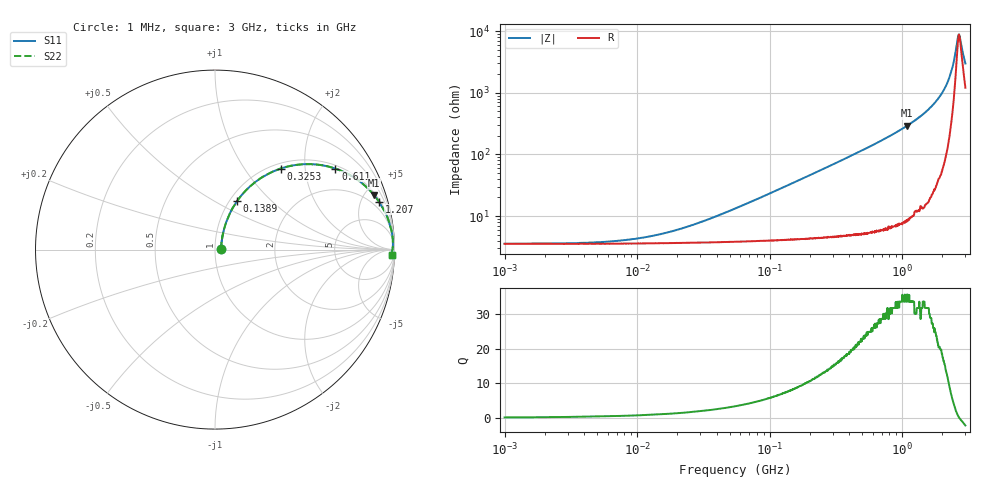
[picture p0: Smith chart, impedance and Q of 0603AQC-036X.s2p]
!s-Parameter Generated by FASTRON Sdn. Bhd.
!FASTRON P/N : 0603AQC-036X
!Keysight Technologies: E4991B_MY54100416_A.01.15
!Date: Thu Jun 25 13:53:48 2026
!Version  :Rev00  Thu Jun 25 13:53:48 2026
!Data & Calibration Information:
!Freq  S11  S21  S12  S22
!PortZ  Port1:50+j0  Port2:50+j0
!When reading reference impedance value at option line is always used.
! Remarks : This data is being provided solely for informational purposes.
# Hz S dB R 50
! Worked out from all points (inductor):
!   1601 points, 1 MHz to 3 GHz, reference 50 ohm
!   read as one part in series: L = 36.6 nH near 49.56 MHz
!   highest Q = 33.8 at 1.086 GHz (marker M1), where L = 42.6 nH
!   self-resonance near 2.687 GHz
!   S11 on the Smith chart (normalised r, x): 1 MHz: 1.07, +0.01; 138.9 MHz: 1.08, +0.64; 325.3 MHz: 1.09, +1.49; 611 MHz: 1.11, +2.89; 1.207 GHz: 1.21, +6.77; 3 GHz: 25, -55
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1000000  -29.30 3.9  -0.30 -0.1  -0.30 -0.1  -29.30 3.9
3804036  -29.00 14.3  -0.30 -0.5  -0.30 -0.5  -29.00 14.3
7588332  -28.20 26.3  -0.31 -1.0  -0.31 -1.0  -28.20 26.3
1.447069e7  -26.30 41.7  -0.31 -1.9  -0.31 -1.9  -26.30 41.7
2.704826e7  -23.00 56.3  -0.33 -3.5  -0.33 -3.5  -23.00 56.3
5.504702e7  -17.90 66.3  -0.39 -7.0  -0.39 -7.0  -17.90 66.3
1.389236e8  -10.60 65.7  -0.74 -16.9  -0.74 -16.9  -10.60 65.7
2.083556e8  -7.62 60.3  -1.19 -24.5  -1.19 -24.5  -7.62 60.3
3.252521e8  -4.72 51.0  -2.17 -35.4  -2.17 -35.4  -4.72 51.0
6.110031e8  -1.85 33.9  -5.06 -53.9  -5.06 -53.9  -1.85 33.9
7.925923e8  -1.14 26.8  -6.92 -61.2  -6.92 -61.2  -1.14 26.8
1.086329e9  -0.56 18.8  -9.83 -69.5  -9.83 -69.5  -0.56 18.8
1.206698e9  -0.43 16.3  -11.00 -72.0  -11.00 -72.0  -0.43 16.3
1.629261e9  -0.18 9.8  -15.40 -78.2  -15.40 -78.2  -0.18 9.8
2.061253e9  -0.08 5.1  -21.00 -81.4  -21.00 -81.4  -0.08 5.1
2.335937e9  -0.07 2.7  -26.60 -79.1  -26.60 -79.1  -0.07 2.7
2.443543e9  -0.07 1.8  -29.90 -74.4  -29.90 -74.4  -0.07 1.8
2.594767e9  -0.09 0.7  -36.40 -49.0  -36.40 -49.0  -0.09 0.7
2.660507e9  -0.10 0.2  -38.80 -17.7  -38.80 -17.7  -0.10 0.2
2.741597e9  -0.11 -0.3  -37.50 23.0  -37.50 23.0  -0.11 -0.3
2.911267e9  -0.12 -1.2  -31.90 57.2  -31.90 57.2  -0.12 -1.2
3e9  -0.12 -1.7  -29.60 64.4  -29.60 64.4  -0.12 -1.7
